(* Logix 5000 AddOnInstructionDefinition export AKD_Stop_Smooth; software revision 19.01 *)

TYPE AKD_Status :   // All connections to the drive ethernet module are established and data is successfully transferring.
STRUCT
   Profile_In_Progress : BOOL;   // Profile Move In Progress
   Block_In_Execution : BOOL;   // Block In Execution
   On_Target_Position : BOOL;   // On Target Position (1=Current Position Equals Last Target Position)
   General_Fault : BOOL;   // General Fault
   Current_Direction : BOOL;   // Current Motor Direction (0=Reverse, 1=Forward)
   Home_Level : BOOL;   // Level of Home Input
   Reg_Level : BOOL;   // Level of Registration Input
   Enable : BOOL;   // State of Enable Output
   Fault_Input_Fault : BOOL;   // Fault Input Active
   Fwd_Limit : BOOL;   // Forward Input Active
   Rev_Limit : BOOL;   // Reverse Input Active
   Positive_Limit : BOOL;   // Positive Software Limit Exceeded
   Negative_Limit : BOOL;   // Negative Software Limit Exceeded
   FE_Fault : BOOL;   // Following Error Fault
   Block_Fault : BOOL;   // Block Execution Fault
   Load_Complete : BOOL;   // Command Message Successfully Loaded
END_STRUCT
END_TYPE

TYPE AKD_Control :   // Send Explicit Message
STRUCT
   Load_Data_Start_Profile : BOOL;   // Load Command Data / Start Profile Move
   Start_Block : BOOL;   // Execute Command block or block chain
   Incremental : BOOL;   // Incremental Position (0=Absolute, 1=Incremental)
   Direction : BOOL;   // Direction in Velocity Mode (0=Reverse, 1=Forward)
   Smooth_Stop : BOOL;   // Smooth / Controlled Stop w/ Deceleration
   Hard_Stop : BOOL;   // Hard / Immediate Stop
   Reg_Arm : BOOL;   // Arm the Registration Input
   Enable : BOOL;   // Enable Output
END_STRUCT
END_TYPE

TYPE AKD_Axis :   // Axis Data:
STRUCT
   Control : AKD_Control;   // Control bits to send to the drive
   Status : AKD_Status;   // Status bits received from the drive
   Input : AB:ETHERNET_MODULE_SINT_64Bytes:I:0;   // Data from the drive
   Output : AB:ETHERNET_MODULE_SINT_64Bytes:O:0;   // Data to the drive
   ResponseMsgType : SINT;   // Response type contained in latest IO response from drive. Used to check for errors
   CommandTimeout : INT;   // Time to allow for command response from drive. Dependent on scan rate and communicaiton rate
   PositionFeedback : DINT;   // Actual Position Value
   VelocityFeedback : DINT;   // Actual Velocity Value
END_STRUCT
END_TYPE

ADD_ON_INSTRUCTION AKD_Stop_Smooth   (* revision 4.0, ExecutePrescan, ExecuteEnableInFalse *)
// Motion Smooth Stop
// Revision note:
// There was a race with the control word smooth stop bit.  I removed the logic in "EnableInFalse" and did the reset as part of the normal logic.
VAR_OUTPUT
   DN : BOOL; {access Read Only, visible}   // Command Successful
   ER : BOOL; {access Read Only, visible}   // Error
END_VAR
VAR_IN_OUT
   Axis : AKD_Axis; {required}
END_VAR
VAR_OUTPUT
   IP : BOOL; {access Read Only, visible}   // In Progress
END_VAR
VAR
   One_SHT : BOOL; {access None}
   Step : DINT; {access None}
END_VAR

ROUTINE EnableInFalse   (* ladder *)
// Enable In False
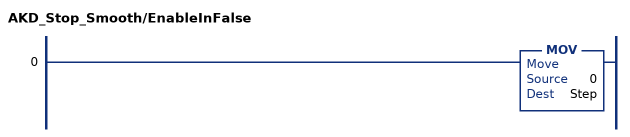
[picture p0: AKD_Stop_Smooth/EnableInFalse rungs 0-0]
   0: MOV(0,Step);
END_ROUTINE

ROUTINE Logic   (* ladder *)
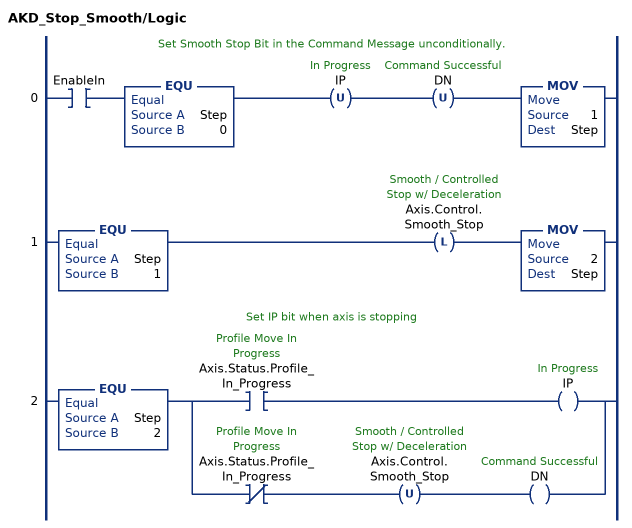
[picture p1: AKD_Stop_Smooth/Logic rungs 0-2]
   // Set Smooth Stop Bit in the Command Message unconditionally.
   0: XIC(EnableIn)EQU(Step,0)OTU(IP)OTU(DN)MOV(1,Step);
   1: EQU(Step,1)OTL(Axis.Control.Smooth_Stop)MOV(2,Step);
   // Set IP bit when axis is stopping
   2: EQU(Step,2)[XIC(Axis.Status.Profile_In_Progress) OTE(IP) ,XIO(Axis.Status.Profile_In_Progress) OTU(Axis.Control.Smooth_Stop) OTE(DN) ];
END_ROUTINE

ROUTINE Prescan   (* ladder *)
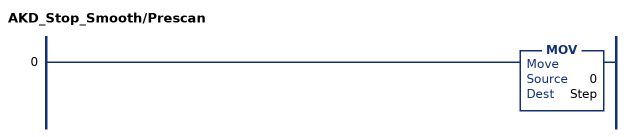
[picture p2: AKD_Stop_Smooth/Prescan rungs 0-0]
   0: MOV(0,Step);
END_ROUTINE
END_ADD_ON_INSTRUCTION
